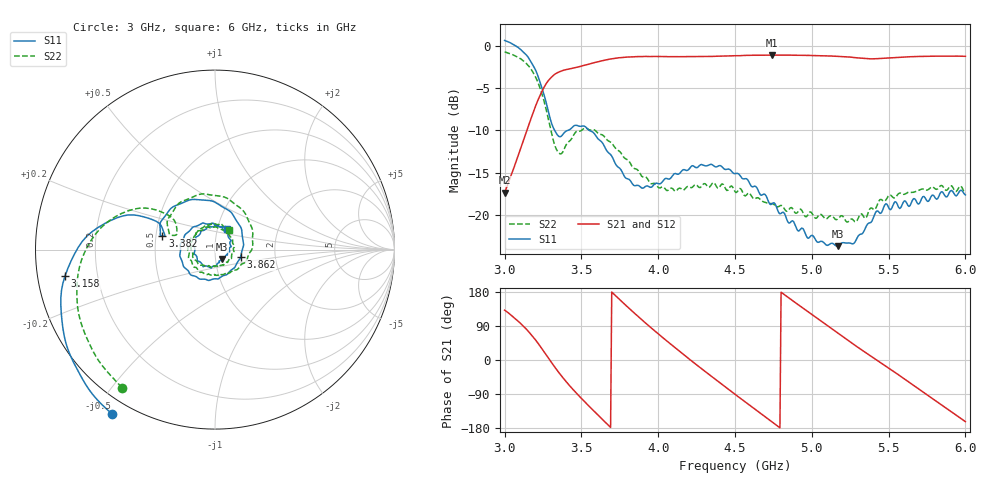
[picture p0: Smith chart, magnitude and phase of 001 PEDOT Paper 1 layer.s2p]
!  04/11/2025  18:25:19
! Ref Plane: 0.000 mm
# MHZ S MA R  50
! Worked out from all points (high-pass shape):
!   401 points, 3 GHz to 6 GHz, reference 50 ohm
!   highest |S21| = -1.05 dB at 4.74 GHz (marker M1); lowest = -17.4 dB at 3 GHz (marker M2)
!   |S21| within 3 dB of the highest: 3.286 GHz to end of sweep
!   lowest |S11| = -23.7 dB at 5.168 GHz (marker M3), VSWR 1.14, Z = 53.6 - j5.7 ohm
!   |S11| at or under -10 dB: 3.326 GHz to 3.41 GHz (84.39 MHz wide, 2.51 % of centre); 3.552 GHz to end of sweep
!   |S22| runs from -20.9 to -0.7 dB; largest |S21 - S12| = 0.012
!   S11 on the Smith chart (normalised r, x): 3 GHz: -0.05, -0.55; 3.158 GHz: 0.08, -0.09; 3.382 GHz: 0.54, +0.09; 3.862 GHz: 1.33, -0.11; 6 GHz: 1.11, +0.26
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3000  1.081 -121.9  0.1349 131.6  0.1357 132.2  0.9265 -124.0
3157.5  0.8481 -170.1  0.3419 74.2  0.342 74.9  0.7612 -172.7
3225  0.6337 166.9  0.4973 40.0  0.4985 40.5  0.5834 161.6
3292.5  0.3844 154.4  0.6369 0.8  0.6384 1.2  0.343 144.2
3382.5  0.3025 165.4  0.7191 -48.2  0.72 -48.0  0.2394 160.7
3502.5  0.3355 140.7  0.763 -102.4  0.7634 -102.2  0.3172 136.5
3690  0.2275 67.3  0.8395 -177.8  0.8399 -177.5  0.2694 56.1
3862.5  0.1494 -16.1  0.8672 117.2  0.8685 117.7  0.1855 -19.6
4005  0.1525 -69.2  0.8677 67.3  0.8691 67.8  0.1443 -62.8
4125  0.1739 -106.0  0.8661 27.5  0.8676 27.9  0.1408 -91.7
4237.5  0.1923 -138.5  0.8674 -9.0  0.8686 -8.3  0.1502 -122.4
4380  0.1923 178.5  0.8719 -53.5  0.8746 -52.9  0.1466 -169.8
4500  0.1753 139.8  0.8782 -90.4  0.8805 -90.0  0.1371 147.1
4612.5  0.1464 101.8  0.8833 -124.6  0.8838 -124.4  0.1269 104.8
4740  0.1159 55.1  0.8858 -163.2  0.8844 -162.8  0.1166 56.6
4860  0.08983 15.2  0.8852 161.0  0.8832 161.5  0.1098 12.3
5002.5  0.07543 -24.1  0.8802 119.2  0.8787 119.6  0.1015 -28.5
5167.5  0.06507 -54.4  0.8714 71.4  0.8699 71.6  0.09408 -74.5
5332.5  0.07784 -79.3  0.8465 24.4  0.8459 24.7  0.09914 -105.8
5505  0.1082 -132.3  0.8518 -22.5  0.8523 -21.8  0.1308 -158.8
5752.5  0.12 138.7  0.8715 -92.4  0.8726 -91.8  0.1401 117.8
6000  0.131 59.5  0.8712 -162.7  0.8718 -162.2  0.1342 54.8
